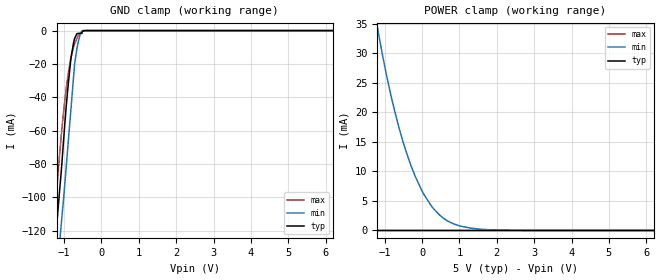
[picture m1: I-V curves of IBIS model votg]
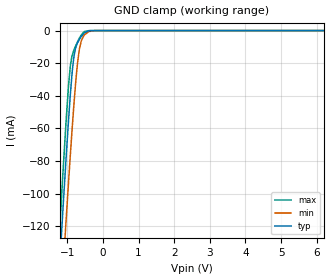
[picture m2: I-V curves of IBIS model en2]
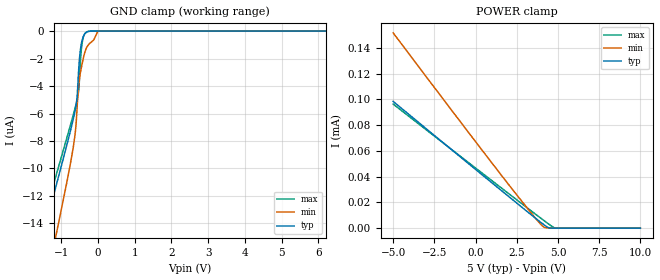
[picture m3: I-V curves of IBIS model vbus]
|Texas Instruments Incorporated
| USB OTG Companion Device with Vbus Over Voltage, Over Current Protection,
| and Four Channel ESD Clamp
| Marketing part#   Digital Voltage Range   Package-type   #pins
| TPD4S214YFFR   4.5V - 5.5V   WCSP-YFF   12
[IBIS Ver]   4.1
[File name]   tpd4s214.ibs
[File Rev]   1.0
[Date]   2/14/2013
[Source]
| Texas Instruments Incorporated.
| Analog-eLab Design Center, HPA
| 12500 TI Blvd
| Dallas, TX -75243
[Notes]   Revision History:
| Rev 1.0: 2/14/2013
| - Initial version of the model
| - Model generated from simulations in TISPICE
| - Model matched to SPICE simulation
| - C_comp although listed in numerical order of value are
|   obtained from varying PVT conditions. For PVT conditions for
|   each specific value refer the buffer description under
|   respective [Model]. IBIS model user is responsible for using
|   appropriate C_comp to simulate for Signal Integrity.
|*  EXCEPTION:   *
|*  - For model vbus, there will be a leakage current in the POWER   *
|*   clamp I-V Table because of the XMMN2 transistor connected to pad.   *
|*  - For model det_fltz, there will be a leakage current in the POWER   *
|*   clamp I-V Table because of the MMP0-MMP3 transistors connected   *
|*   to pad.   *
|*  - For model votg, there will be a leakage current in the power clamp   *
|*   I-V Table because of the BJT in the buffercell connected to pad.   *
|*  - For model votg, there will be a leakage current in the ground clamp   *
|*   I-V Table because of the pull down transistors in esd connected to pad *
|*  - For model adj , there will be a leakage current in the power clamp   *
|*   I-V Table because of the transistors in buffercell connected to pad.   *
|*  - For model dpm, there will be a leakage current in the power clamp   *
|*   I-V Table because of the diodes connected to pad.   *
[Disclaimer]
| This model is designed as an aid for customers of Texas Instruments.
| TI and its licensors and suppliers make no warranties, either expressed
| or implied, with respect to this  model, including the warranties of
| merchantability or fitness for a particular purpose. The model is
| provided solely on an "as is" basis. The entire risk as to its quality
| and performance is with the customer.
[Copyright]
(C) Copyright 2013 Texas Instruments Incorporated.All rights reserved.
|   TPD4S214
[Component]   TPD4S214
[Manufacturer]   TI
[Package]   |12 WCSP - YFF package
|   typ   min   max
R_pkg   0.00500   0.00500   0.00500
L_pkg   0.20000nH   0.20000nH   0.20000nH
C_pkg   0.60000pF   0.60000pF   0.60000pF
[Pin]  signal_name   model_name   R_pin   L_pin   C_pin
A1   VOTG_IN   votg   0.00500   0.20000nH  0.60000pF
A2   DET   det_fltz   0.00500   0.20000nH  0.60000pF
A3   VBUS   vbus   0.00500   0.20000nH  0.60000pF
B1   VOTG_IN   votg   0.00500   0.20000nH  0.60000pF
B2   _FLT   det_fltz   0.00500   0.20000nH  0.60000pF
B3   VBUS   vbus   0.00500   0.20000nH  0.60000pF
C1   EN   en2   0.00500   0.20000nH  0.60000pF
C2   GND   GND   0.00500   0.20000nH  0.60000pF
C3   ID   dpm   0.00500   0.20000nH  0.60000pF
D1   ADJ   adj   0.00500   0.20000nH  0.60000pF
D2   D-   dpm   0.00500   0.20000nH  0.60000pF
D3   D+   dpm   0.00500   0.20000nH  0.60000pF
| Models and submodels in the file (6): votg (Input), en2 (Input), vbus (Input), adj (Input), dpm (Input), det_fltz (Open_drain)
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|   votg Model
[Model]   votg
Model_type   Input
Vinl = 0.4
Vinh = 1.2
|   typ   min   max
|   (nom PVT)   (fast PVT)   (slow PVT)
C_comp   3.962e-11   3.771e-11   4.277e-11
| Where nom  PVT is Nominal Process, 5V, 27C
|   Fast PVT is Strong Process,  5.5V, -40C
|   Slow PVT is Weak Process,   4.5V, 125C
[Voltage Range]   5   4.5   5.5
|Junction Temperature
[Temperature Range]   27   125   -40
[Power Clamp Reference]   5   4.5   5.5
[GND Clamp Reference]   0   0   0
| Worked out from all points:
|   GND clamp passes 1 mA (typ) near -0.52 V on its own axis
[GND Clamp]
|   Voltage   I(typ)   I(min)   I(max)
-5V       -1.94A     -1.924A    -1.971A
-1.571V   -247.5mA   -268mA     -239.6mA
-1.252V   -132.9mA   -163.8mA   -113.8mA
-1.161V   -107.3mA   -138.6mA   -86.09mA
-1.135V   -100.3mA   -131.5mA   -78.72mA
-1.073V   -84.28mA   -115.8mA   -62.84mA
-940mV    -45.28mA   -81.39mA   -34.47mA
-814.5mV  -16.68mA   -47.05mA   -16.38mA
-715.5mV  -4.685mA   -19.85mA   -7.707mA
-617mV    -1.702mA   -6.545mA   -2.908mA
-513.5mV  -828.6uA   -751.5nA   -540.1uA
10V       0A         0A         0A
[POWER Clamp]
|   Voltage   I(typ)   I(min)   I(max)
-5V       281.4uA    381.5mA    275.4uA
-1.252V   0A         36.54mA    0A
-1.153V   0A         32.92mA    0A
-837.5mV  0A         23.01mA    0A
-611mV    0A         17.27mA    0A
-392mV    0A         12.71mA    0A
-182mV    0A         9.167mA    0A
62.5mV    0A         5.981mA    0A
310mV     0A         3.674mA    0A
881.5mV   0A         1.032mA    0A
2.165V    0A         44.13uA    0A
10V       0A         0A         0A
|   en2 Model
[Model]   en2
Model_type   Input
Vinl = 0.4
Vinh = 1.2
|   typ   min   max
|   (nom PVT)   (fast PVT)   (slow PVT)
C_comp   1.352e-12   1.322e-12   1.397e-12
| Where nom  PVT is Nominal Process, 5V, 27C
|   Fast PVT is Strong Process,  5.5V, -40C
|   Slow PVT is Weak Process,   4.5V, 125C
[Voltage Range]   5   4.5   5.5
|Junction Temperature
[Temperature Range]   27   125   -40
[Power Clamp Reference]   5   4.5   5.5
[GND Clamp Reference]   0   0   0
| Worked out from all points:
|   GND clamp passes 1 mA (typ) near -0.48 V on its own axis
[GND Clamp]
|   Voltage   I(typ)   I(min)   I(max)
-5V       -1.713A    -1.689A    -1.74A
-1.249V   -156.9mA   -193.4mA   -136mA
-1.128V   -111.9mA   -149.7mA   -89.65mA
-1.036V   -78.9mA    -117.2mA   -56.29mA
-968.5mV  -56.28mA   -94.31mA   -34.88mA
-919mV    -40.83mA   -77.93mA   -22.79mA
-825mV    -17.93mA   -48.66mA   -12.66mA
-750mV    -9.578mA   -28.4mA    -8.653mA
-666mV    -5.671mA   -12.26mA   -4.873mA
-517.5mV  -1.354mA   -2.604mA   -604.5uA
-221mV    -615.1nA   -15.94uA   -11.73nA
10V       0A         0A         0A
[POWER Clamp]
|   Voltage   I(typ)   I(min)   I(max)
-5V       0A         0A         0A
0V        0A         0A         0A
10V       0A         0A         0A
|   vbus Model
[Model]   vbus
Model_type   Input
Vinl = 0.4
Vinh = 1.2
|   typ   min   max
|   (nom PVT)   (fast PVT)   (slow PVT)
C_comp   6.001e-11   5.821e-11   6.190e-11
| Where nom  PVT is Nominal Process, 5V, 27C
|   Fast PVT is Strong Process,  5.5V, -40C
|   Slow PVT is Weak Process,   4.5V, 125C
[Voltage Range]   5   4.5   5.5
|Junction Temperature
[Temperature Range]   27   125   -40
[Power Clamp Reference]   5   4.5   5.5
[GND Clamp Reference]   0   0   0
[GND Clamp]
|   Voltage   I(typ)   I(min)   I(max)
-5V       -49.9uA    -63.81uA   -46.34uA
-1.249V   -12.38uA   -16.26uA   -11.53uA
-1.036V   -10.22uA   -13.51uA   -9.547uA
-747.5mV  -7.256uA   -9.631uA   -6.843uA
-610mV    -5.631uA   -7.228uA   -5.485uA
-565mV    -4.741uA   -5.501uA   -4.978uA
-534mV    -3.281uA   -4.273uA   -4.541uA
-457mV    -1.018uA   -2.747uA   -1.51uA
-396.5mV  -396.4nA   -1.971uA   -440.5nA
-303mV    -69.99nA   -1.169uA   -52.39nA
-500uV    0A         0A         0A
10V       0A         0A         0A
[POWER Clamp]
|   Voltage   I(typ)   I(min)   I(max)
-5V       98.47uA    151.7uA    96.4uA
1.523V    29.69uA    41.87uA    31.66uA
3.582V    8.326uA    8.531uA    11.42uA
4.099V    3.146uA    1.321uA    6.403uA
4.215V    2.046uA    476.9nA    5.291uA
4.441V    266.1nA    185.5nA    3.155uA
4.834V    0A         0A         112.4nA
10V       0A         0A         0A
